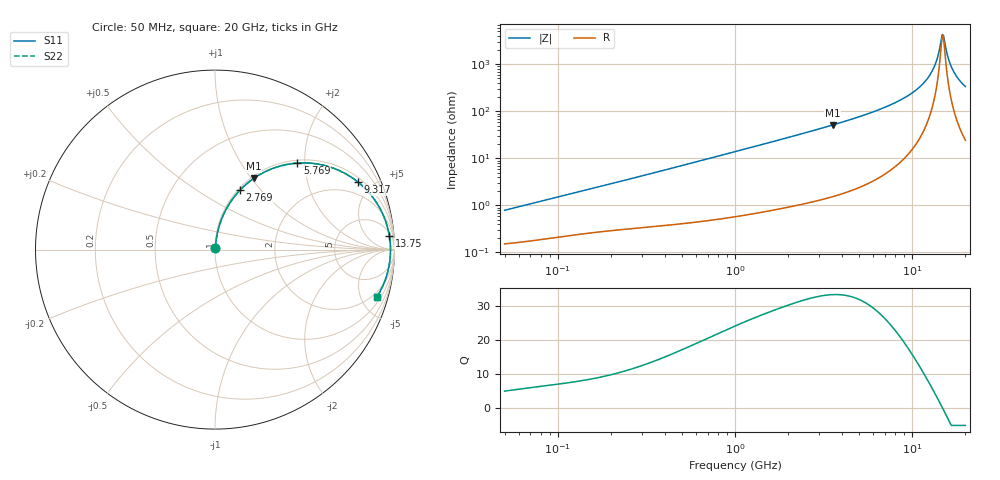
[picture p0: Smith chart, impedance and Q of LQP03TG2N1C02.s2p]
!Murata Part Number: LQP03TG2N1C02
!These Parameters are Measured in Series Mode Connection
!  o--[Z]--o
!Port1  Port2
!  o-------o
!Freq. Start=50[MHz] Stop=20[GHz], 401[Steps]
# Hz S RI R 50
!Freq.(Hz) S11(Real) S11(Imag) S21(Real) S21(Imag) S12(Real) S12(Imag) S22(Real) S22(Imag)
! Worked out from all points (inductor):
!   401 points, 50 MHz to 20 GHz, reference 50 ohm
!   read as one part in series: L = 2.44 nH near 51.52 MHz
!   highest Q = 33.4 at 3.572 GHz (marker M1), where L = 2.29 nH
!   self-resonance near 14.82 GHz
!   S11 on the Smith chart (normalised r, x): 50 MHz: 1.00, +0.02; 2.769 GHz: 1.02, +0.78; 5.769 GHz: 1.06, +1.84; 9.317 GHz: 1.23, +4.13; 13.75 GHz: 8, +23; 20 GHz: 1.49, -6.72
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5e7  0.00158 0.00772  0.9984 -0.00772  0.9984 -0.00772  0.00158 0.00772
1.364002e8  0.00286 0.02  0.9971 -0.02  0.9971 -0.02  0.00286 0.02
3.721004e8  0.00635 0.052  0.9937 -0.052  0.9937 -0.052  0.00635 0.052
1e9  0.0243 0.1348  0.9757 -0.1348  0.9757 -0.1348  0.0243 0.1348
2.728004e9  0.1365 0.3283  0.8635 -0.3283  0.8635 -0.3283  0.1365 0.3283
2.769174e9  0.1401 0.3321  0.8599 -0.3321  0.8599 -0.3321  0.1401 0.3321
3.572216e9  0.2167 0.3973  0.7833 -0.3973  0.7833 -0.3973  0.2167 0.3973
5.769027e9  0.4594 0.4821  0.5406 -0.4821  0.5406 -0.4821  0.4594 0.4821
7.442007e9  0.6376 0.4611  0.3624 -0.4611  0.3624 -0.4611  0.6376 0.4611
9.316812e9  0.7976 0.3754  0.2024 -0.3754  0.2024 -0.3754  0.7976 0.3754
1.066139e10  0.8798 0.2905  0.1202 -0.2905  0.1202 -0.2905  0.8798 0.2905
1.183995e10  0.9296 0.209  0.0704 -0.209  0.0704 -0.209  0.9296 0.209
1.295331e10  0.9594 0.1308  0.0406 -0.1308  0.0406 -0.1308  0.9594 0.1308
1.375312e10  0.9716 0.0757  0.0284 -0.0757  0.0284 -0.0757  0.9716 0.0757
1.460232e10  0.9775 0.0193  0.0225 -0.0193  0.0225 -0.0193  0.9775 0.0193
1.482269e10  0.9779 0.00512  0.0221 -0.00512  0.0221 -0.00512  0.9779 0.00512
1.504638e10  0.9779 -0.0091  0.0221 0.0091  0.0221 0.0091  0.9779 -0.0091
1.527346e10  0.9775 -0.0233  0.0225 0.0233  0.0225 0.0233  0.9775 -0.0233
1.621653e10  0.9718 -0.0798  0.0282 0.0798  0.0282 0.0798  0.9718 -0.0798
1.696185e10  0.9632 -0.1214  0.0368 0.1214  0.0368 0.1214  0.9632 -0.1214
1.828096e10  0.9412 -0.1881  0.0588 0.1881  0.0588 0.1881  0.9412 -0.1881
2e10  0.9031 -0.2618  0.0969 0.2618  0.0969 0.2618  0.9031 -0.2618
